FUNCTION_BLOCK Example03_groups //2x1 flyways w/ 2 xbots - async,async velocity, create group,block&release group buffer, bond&unbond group
VAR_INPUT
	Execute : BOOL;
END_VAR
VAR_OUTPUT
	Done : BOOL;
END_VAR
VAR_IN_OUT
	PM_Controller : PMControllerType;	// the planar motor controller to use
END_VAR
VAR
	xbotID_array78 : ARRAY[0..77] OF USINT;
	PosX_array78 : ARRAY[0..77] OF REAL;
	PosY_array78 : ARRAY[0..77] OF REAL;
	PMC_AutoDrivingMotion1 : PMC_AutoDrivingMotion;
	xbotID_array32 : ARRAY[0..31] OF USINT;
	PMC_CreateXbotGroup1 : PMC_CreateXbotGroup;
	PMC_BlockXbotGroup1 : PMC_BlockXbotGroup;
	PMC_XYMotion1 : PMC_XYMotion;
	PMC_XYMotion2 : PMC_XYMotion;
	PMC_BlockXbotGroup2 : PMC_BlockXbotGroup;
	PMC_XYMotion3 : PMC_XYMotion;
	PMC_AutoDrivingMotionVelocity1 : PMC_AutoDrivingMotionVelocity;
	PMC_BondXbotGroup1 : PMC_BondXbotGroup;
	PMC_XYMotion4 : PMC_XYMotion;
	PMC_XYMotion5 : PMC_XYMotion;
	PMC_XYMotion6 : PMC_XYMotion;
	PMC_BondXbotGroup2 : PMC_BondXbotGroup;
	PMC_XYMotion7 : PMC_XYMotion;
	PMC_DeleteXbotGroup1 : PMC_DeleteXbotGroup;
END_VAR

//2x1 flyways w/ 2 xbots - async,async velocity, create group,block&release group buffer, bond&unbond group

//async move to 60,60 and 60,180
xbotID_array78[0] := 1;xbotID_array78[1] := 2;
PosX_array78[0] := 0.06;PosX_array78[1] := 0.06;
PosY_array78[0] := 0.06;PosY_array78[1] := 0.18;
PMC_AutoDrivingMotion1(Execute := Execute,nXbots := 2,RoutingType := 0,ZoneID := 0,XbotID := xbotID_array78,PosX := PosX_array78,PosY := PosY_array78,PM_Controller := PM_Controller);

// create group 1 w/ xbots 1 and 2
xbotID_array32[0] := 1;xbotID_array32[1] := 2;
PMC_CreateXbotGroup1(Execute := PMC_AutoDrivingMotion1.Done,GroupID := 1,nXbots := 2,XbotID := xbotID_array32,PM_Controller := PM_Controller);

//block buffer for group 1
PMC_BlockXbotGroup1(Execute := PMC_CreateXbotGroup1.Done,GroupID := 1,IsBlock := TRUE,PM_Controller := PM_Controller);

// load command to move xbot 1 to 420,60
PMC_XYMotion1(Execute := PMC_BlockXbotGroup1.Done,cmdLB := 4,XbotID := 1,Mode := 0,Type_ := 0,PosX := 0.42,PosY := 0.06,EndVel := 0,MaxVel := 1,MaxAcc := 10,PM_Controller := PM_Controller);

//load command to move xbot 2 to 420,180
PMC_XYMotion2(Execute := PMC_XYMotion1.Ack,cmdLB := 5,XbotID := 2,Mode := 0,Type_ := 0,PosX := 0.42,PosY := 0.18,EndVel := 0,MaxVel := 1,MaxAcc := 10,PM_Controller := PM_Controller);

//release buffer for group 1
PMC_BlockXbotGroup2(Execute := PMC_XYMotion2.Ack,GroupID := 1,IsBlock := FALSE,PM_Controller := PM_Controller);

//move xbot 1 to 60,60
PMC_XYMotion3(Execute := PMC_BlockXbotGroup2.Done AND PMC_XYMotion2.Done,cmdLB := 7,XbotID := 1,Mode := 0,Type_ := 0,PosX := 0.06,PosY := 0.06,EndVel := 0,MaxVel := 1,MaxAcc := 10,PM_Controller := PM_Controller);

// async move to 180,60 and 180,180 at user set speed and acceleration
xbotID_array78[0] := 1;xbotID_array78[1] := 2;
PosX_array78[0] := 0.180;PosX_array78[1] := 0.060;
PosY_array78[0] := 0.180;PosY_array78[1] := 0.180;
PMC_AutoDrivingMotionVelocity1(Execute := PMC_XYMotion3.Done,nXbots := 2,RoutingType := 0,ZoneID := 0,XbotID := xbotID_array78,PosX := PosX_array78,PosY := PosY_array78,MaxVel := 2,MaxAcc := 20,PM_Controller := PM_Controller);

// bond xbots in group 1
PMC_BondXbotGroup1(Execute := PMC_AutoDrivingMotionVelocity1.Done,GroupID := 1,IsBond := TRUE,Mode := 0,PM_Controller := PM_Controller);

// move xbot 1 to 420,60
PMC_XYMotion4(Execute := PMC_BondXbotGroup1.Done,cmdLB := 10,XbotID := 1,Mode := 0,Type_ := 0,PosX := 0.42,PosY := 0.06,EndVel := 0,MaxVel := 1,MaxAcc := 10,PM_Controller := PM_Controller);

//move xbot 2 to 300,180
PMC_XYMotion5(Execute := PMC_XYMotion4.Done,cmdLB := 11,XbotID := 2,Mode := 0,Type_ := 0,PosX := 0.3,PosY := 0.18,EndVel := 0,MaxVel := 1,MaxAcc := 10,PM_Controller := PM_Controller);

//move xbot 1 to 180,60
PMC_XYMotion6(Execute := PMC_XYMotion5.Done,cmdLB := 12,XbotID := 1,Mode := 0,Type_ := 0,PosX := 0.18,PosY := 0.06,EndVel := 0,MaxVel := 1,MaxAcc := 10,PM_Controller := PM_Controller);

//unbond xbots in group 1
PMC_BondXbotGroup2(Execute := PMC_XYMotion6.Done,GroupID := 1,IsBond := FALSE,Mode := 0,PM_Controller := PM_Controller);

//move xbot 1 to 180,180
PMC_XYMotion7(Execute := PMC_BondXbotGroup2.Done,cmdLB := 14,XbotID := 1,Mode := 0,Type_ := 0,PosX := 0.18,PosY := 0.18,EndVel := 0,MaxVel := 1,MaxAcc := 10,PM_Controller := PM_Controller);

//delete group 1
PMC_DeleteXbotGroup1(Execute := PMC_XYMotion7.Done,GroupID := 1,PM_Controller := PM_Controller);
	
Done := PMC_DeleteXbotGroup1.Done;

END_FUNCTION_BLOCK
